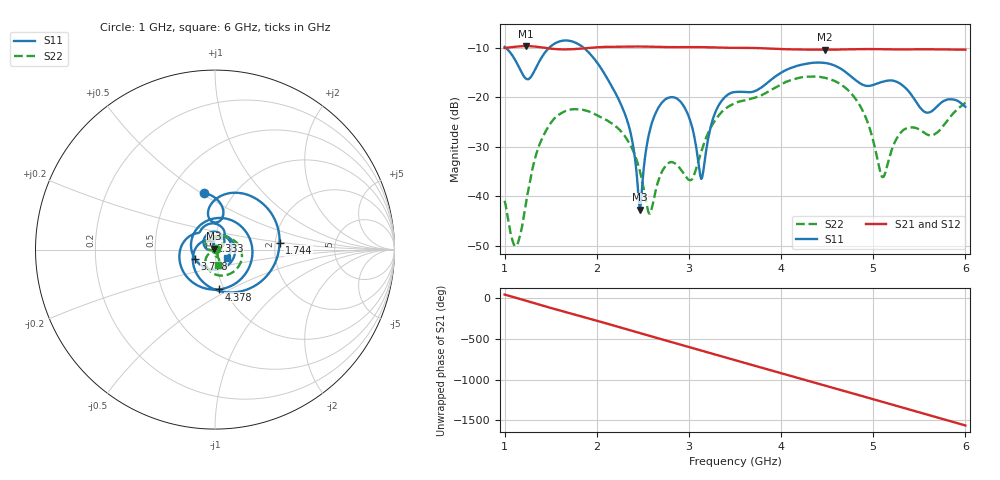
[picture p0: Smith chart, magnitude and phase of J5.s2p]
!Agilent Technologies,E8364B,MY43040528,A.07.50.67
!Agilent E8364B: A.07.50.67
!Date: Sunday, March 01, 2026 15:25:27
!Correction: S11(Full 2 Port(1,2))
!S21(Full 2 Port(1,2))
!S12(Full 2 Port(1,2))
!S22(Full 2 Port(1,2))
!S2P File: Measurements: S11, S21, S12, S22:
# Hz S  dB  R 50
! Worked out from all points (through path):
!   451 points, 1 GHz to 6 GHz, reference 50 ohm
!   highest |S21| = -9.70 dB at 1.233 GHz (marker M1); lowest = -10.4 dB at 4.478 GHz (marker M2)
!   group delay of S21, straight-line fit = 892 ps
!   lowest |S11| = -42.7 dB at 2.467 GHz (marker M3), VSWR 1.01, Z = 49.5 + j0.52 ohm
!   |S11| at or under -10 dB: 1.01 GHz to 1.485 GHz (475.5 MHz wide, 38.1 % of centre); 1.856 GHz to end of sweep
!   |S22| runs from -50.1 to -15.8 dB; largest |S21 - S12| = 0.0014
!   S11 on the Smith chart (normalised r, x): 1 GHz: 0.73, +0.51; 1.744 GHz: 2.11, +0.18; 2.333 GHz: 0.94, +0.10; 3.778 GHz: 0.79, -0.08; 4.378 GHz: 0.94, -0.44; 6 GHz: 1.14, -0.10
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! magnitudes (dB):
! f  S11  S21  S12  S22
! 1 GHz  -9.9  -10.1  -10.1  -41.0
! 1.122 GHz  -12.8  -9.8  -9.9  -50.0
! 1.233 GHz  -16.3  -9.7  -9.7  -41.3
! 1.433 GHz  -11.1  -10.0  -10.1  -27.4
! 1.744 GHz  -8.8  -10.3  -10.3  -22.5
! 1.844 GHz  -9.8  -10.2  -10.2  -22.6
! 2.333 GHz  -24.9  -9.8  -9.8  -28.7
! 2.467 GHz  -42.7  -9.8  -9.8  -34.9
! 2.567 GHz  -27.5  -9.8  -9.8  -43.5
! 2.667 GHz  -22.2  -9.9  -9.9  -37.0
! 2.933 GHz  -21.5  -9.9  -9.9  -35.2
! 3.133 GHz  -36.5  -9.9  -9.9  -31.1
! 3.289 GHz  -23.0  -10.0  -10.0  -24.6
! 3.5 GHz  -19.0  -10.1  -10.1  -21.2
! 3.778 GHz  -18.2  -10.1  -10.1  -19.7
! 4.344 GHz  -13.1  -10.4  -10.4  -15.8
! 4.378 GHz  -13.0  -10.4  -10.4  -15.8
! 4.478 GHz  -13.1  -10.4  -10.5  -16.1
! 4.856 GHz  -17.2  -10.3  -10.3  -21.7
! 5.1 GHz  -16.9  -10.3  -10.4  -36.2
! 5.167 GHz  -16.7  -10.4  -10.4  -32.8
! 6 GHz  -22.0  -10.4  -10.4  -21.1
